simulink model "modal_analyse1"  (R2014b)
settings: Solver=ode4  StartTime=0.0  StopTime=20.0  MaxStep=0.001  RelTol=1e-3
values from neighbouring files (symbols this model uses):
  A = [-c1/m1, -k1/m1, c1/m1, k1/m1    [impuls_antw_zustand_1.m]    (also in modal_analyse_1.m; uebertragung_mechanik_1.m; uebertragung_zustand_1.m = [0,0,1/C1,-1/C1;0,-1/(C2*R2),0,1/C2;       -1/L1, 0 -Rg/L1, )
  B = [0, 0, 1/m2, 0]'    [impuls_antw_zustand_1.m]    (also in modal_analyse_1.m; uebertragung_mechanik_1.m; uebertragung_zustand_1.m = [0,0,1/L1,0]')
  C = [0 1 0 0;0 0 0 1]    [impuls_antw_zustand_1.m]    (also in impuls_antwort_1.m = 1e-07; impuls_antwort_2.m = 1e-07; impuls_antwort_3.m = 1e-07; impuls_antwort_4.m = 1e-07)
  D = zeros(2,1)    [impuls_antw_zustand_1.m]    (also in modal_analyse_1.m = zeros(4,1); uebertragung_mechanik_1.m = zeros(4,1); uebertragung_zustand_1.m = zeros(4,1))
  selekt1 = [0,0,0,1]    [modal_analyse_1.m]
  selekt2 = [0,0,1,0]    [modal_analyse_1.m]
  selekt3 = [0,1,0,0]    [modal_analyse_1.m]
  selekt4 = [1,0,0,0]    [modal_analyse_1.m]

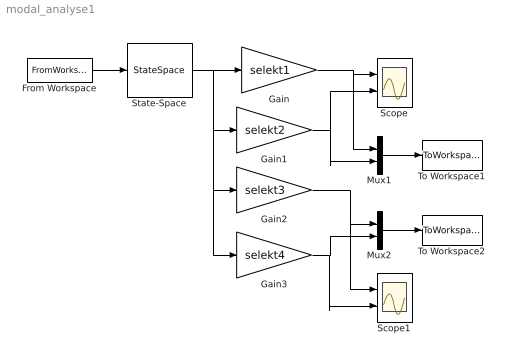
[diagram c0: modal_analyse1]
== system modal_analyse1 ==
  From Workspace : FromWorkspace  VariableName=[t', ug_puls']  SampleTime=0
  Gain : Gain  Gain=selekt1  Multiplication=Matrix(K*u)
  Gain1 : Gain  Gain=selekt2  Multiplication=Matrix(K*u)
  Gain2 : Gain  Gain=selekt3  Multiplication=Matrix(K*u)
  Gain3 : Gain  Gain=selekt4  Multiplication=Matrix(K*u)
  Mux1 : Mux  Inputs=2
  Mux2 : Mux  Inputs=2
  Scope : Scope  NumInputPorts=2
  Scope1 : Scope  NumInputPorts=2
  State-Space : StateSpace  A=A  B=B  C=C  D=D  X0=0
  To Workspace1 : ToWorkspace  VariableName=simout  SaveFormat=Timeseries  SampleTime=-1
  To Workspace2 : ToWorkspace  VariableName=simout1  SaveFormat=Timeseries  SampleTime=-1
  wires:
  Mux1/1 -> To Workspace1/1
  From Workspace/1 -> State-Space/1
  State-Space/1 -> Gain3/1, Gain2/1, Gain1/1, Gain/1
  Gain/1 -> Mux1/1, Scope/1
  Gain1/1 -> Scope/2, Mux1/2
  Gain3/1 -> Scope1/2, Mux2/2
  Gain2/1 -> Scope1/1, Mux2/1
  Mux2/1 -> To Workspace2/1
